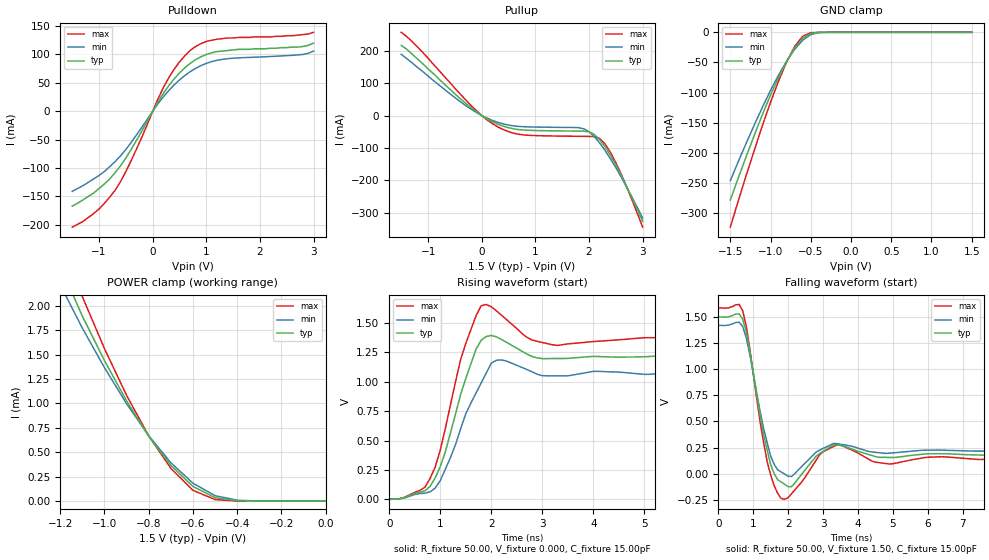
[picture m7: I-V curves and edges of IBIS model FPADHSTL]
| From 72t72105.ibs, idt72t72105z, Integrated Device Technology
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|   Model FPADHSTL
[Model]   FPADHSTL
Model_type   3-state
Polarity   Non-Inverting
Enable   Active-High
Vmeas =  0.750V
C_comp   3.00pF   NA   NA
[Temperature Range]   25.00   85.00   -40.00
[Voltage Range]   1.50V   1.40V   1.60V
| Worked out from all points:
|   slope of the pulldown table from 0 to 0.225 V, typ, clamps not added: 6.42 ohm
|   slope of the pullup table from 0 to 0.225 V, typ, clamps not added: 10.7 ohm
|   GND clamp passes 1 mA (typ) near -0.45 V on its own axis
|   POWER clamp passes 1 mA (typ) near -0.89 V on its own axis
|   rising waveform, R_fixture 50.00, V_fixture 0.000, C_fixture 15.00pF: 20-80 % time 495ps typ, 592ps min, 448ps max; typ from 0 V to 1.21 V
|   falling waveform, R_fixture 50.00, V_fixture 1.50, C_fixture 15.00pF: 20-80 % time 391ps typ, 404ps min, 375ps max; typ from 1.5 V to 0.183 V
[Pulldown]
| voltage   I(typ)   I(min)   I(max)
-1.5V     -167mA     -141mA     -204mA
-1.3V     -156mA     -131mA     -194mA
-1V       -136mA     -113mA     -172mA
-700mV    -108mA     -88.57mA   -139mA
-400mV    -66.98mA   -54.66mA   -86.64mA
200mV     31.71mA    25.58mA    41.77mA
400mV     57.04mA    46.47mA    74.01mA
700mV     84.35mA    69.78mA    107mA
1V        100mA      84.36mA    123mA
1.2V      105mA      89.75mA    127mA
2.7V      113mA      99.15mA    134mA
3V        120mA      106mA      139mA
[Pullup]
| voltage   I(typ)   I(min)   I(max)
-1.5V     217mA      189mA      257mA
-1.1V     160mA      136mA      195mA
-300mV    37.97mA    30.98mA    48.44mA
0V        0A         -10pA      30pA
300mV     -26.66mA   -21.07mA   -35.09mA
800mV     -45.1mA    -34.75mA   -60.27mA
1.9V      -48.49mA   -40.9mA    -64.4mA
2.1V      -58.61mA   -65.6mA    -65.33mA
2.2V      -74.81mA   -85.33mA   -71.21mA
2.3V      -96.98mA   -108mA     -88.2mA
2.5V      -153mA     -161mA     -146mA
3V        -327mA     -317mA     -345mA
[GND_clamp]
| voltage   I(typ)   I(min)   I(max)
-1.5V     -278mA     -246mA     -323mA
-1.3V     -205mA     -183mA     -236mA
-1.1V     -136mA     -124mA     -154mA
-1V       -104mA     -96.2mA    -116mA
-900mV    -74.56mA   -70.77mA   -80.61mA
-800mV    -48.24mA   -47.88mA   -49.04mA
-700mV    -26.16mA   -28.23mA   -23.28mA
-600mV    -10.07mA   -12.98mA   -6.406mA
-500mV    -2.002mA   -3.724mA   -655uA
-400mV    -177uA     -538uA     -28.11uA
1.5V      15.11nA    22.17nA    15nA
[POWER_clamp]
| voltage   I(typ)   I(min)   I(max)
-1.5V     8.542mA    5.787mA    13.11mA
-1.2V     2.409mA    2.216mA    2.73mA
-1.1V     1.896mA    1.773mA    2.096mA
-1V       1.44mA     1.368mA    1.563mA
-900mV    1.027mA    998uA      1.084mA
-800mV    665uA      671uA      669uA
-700mV    367uA      394uA      337uA
-600mV    151uA      184uA      111uA
-500mV    35.56uA    56.06uA    16.17uA
-400mV    4.035uA    9.223uA    1.078uA
0V        15.11nA    18.77nA    16nA
[Ramp]
| variable   typ   min   max
dV/dt_r   0.74/0.27n   0.65/0.33n   0.83/0.25n
dV/dt_f   0.80/0.16n   0.73/0.17n   0.88/0.13n
R_load = 50.00
[Rising Waveform]
R_fixture = 50.00
V_fixture = 0.000
C_fixture = 15.00pF
R_dut = 0.75
L_dut = 8.10nH
C_dut = 0.53pF
| time   V(typ)   V(min)   V(max)
0s        0V         0V         0V
600ps     59.7mV     49.23mV    75.59mV
800ps     109mV      63.46mV    177mV
1ns       277mV      159mV      418mV
1.4ns     893mV      601mV      1.189V
1.8ns     1.351V     988mV      1.645V
2.1ns     1.381V     1.182V     1.602V
2.7ns     1.234V     1.103V     1.376V
3.3ns     1.197V     1.05V      1.308V
9.9ns     1.214V     1.076V     1.358V
[Falling Waveform]
R_fixture = 50.00
V_fixture = 1.50
C_fixture = 15.00pF
R_dut = 0.75
L_dut = 8.10nH
C_dut = 0.53pF
| time   V(typ)   V(min)   V(max)
0s        1.5V       1.419V     1.586V
700ps     1.477V     1.408V     1.558V
1.4ns     229mV      299mV      118mV
1.6ns     1.523mV    91.43mV    -114mV
1.8ns     -78.08mV   18.36mV    -235mV
2.1ns     -123mV     -25.96mV   -190mV
2.9ns     192mV      226mV      181mV
3.4ns     278mV      288mV      277mV
4.9ns     156mV      197mV      93.45mV
9.9ns     183mV      219mV      144mV
